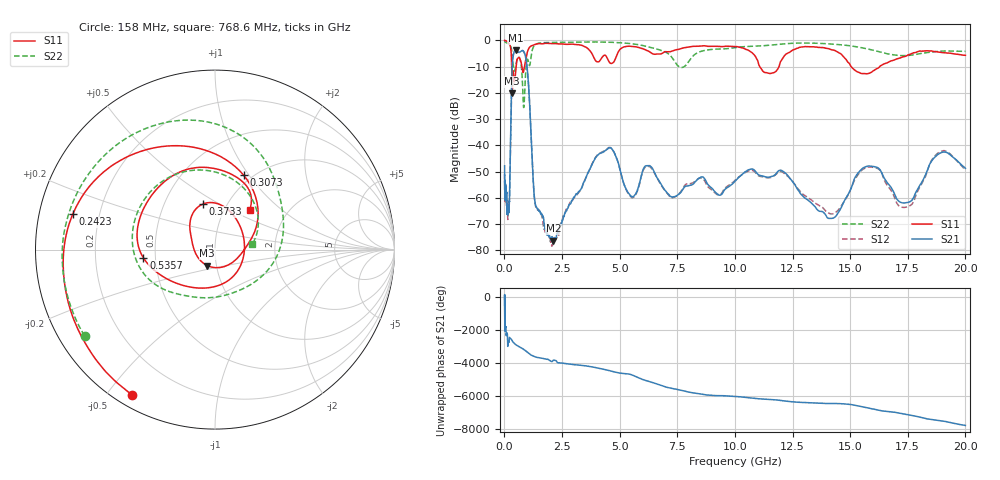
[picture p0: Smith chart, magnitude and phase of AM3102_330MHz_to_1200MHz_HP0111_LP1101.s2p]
! Date/Time: Tue, Sep 11, 2018 5:16 PM
! Network Analyzer: Agilent Technologies E8362B Rev: A.07.50.63
! Sweep from 0.010 to 20.000 GHz, 1601 Points, Sweep Type: LOG
! Power Supply: 4.949 V, 0.001 A
# Hz S DB R 50
!freq MagS11 AngS11 MagS21 AngS21 MagS12 AngS12 MagS22 AngS22
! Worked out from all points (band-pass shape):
!   1601 points, 10 MHz to 20 GHz, reference 50 ohm
!   highest |S21| = -3.69 dB at 491.8 MHz (marker M1); lowest = -76.3 dB at 2.124 GHz (marker M2)
!   |S21| within 3 dB of the highest: 368.5 MHz to 930.7 MHz (562.2 MHz wide, 86.6 % of centre)
!   lowest |S11| = -20.1 dB at 341.1 MHz (marker M3), VSWR 1.22, Z = 45.1 - j8.07 ohm
!   |S11| at or under -10 dB: 317.2 MHz to 509.5 MHz (192.2 MHz wide, 46.5 % of centre); 11.08 GHz to 11.91 GHz (831.3 MHz wide, 7.23 % of centre); 15.04 GHz to 16.28 GHz (1.234 GHz wide, 7.88 % of centre)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
!   |S22| runs from -25.6 to -0.3 dB; largest |S21 - S12| = 0.011
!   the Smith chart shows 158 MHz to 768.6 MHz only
!   S11 on the Smith chart (normalised r, x): 158 MHz: 0.05, -0.58; 242.3 MHz: 0.10, +0.12; 307.3 MHz: 0.92, +0.94; 373.3 MHz: 0.77, +0.42; 535.7 MHz: 0.43, -0.05; 768.6 MHz: 1.31, +0.64
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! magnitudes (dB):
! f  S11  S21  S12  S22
! 10 MHz  0.0  -47.8  -51.5  -0.3
! 35.55 MHz  0.0  -58.7  -59.0  -0.6
! 126.4 MHz  -0.4  -66.2  -65.6  -1.1
! 158 MHz  -0.6  -64.0  -64.8  -1.2
! 242.3 MHz  -1.8  -51.1  -51.2  -1.7
! 307.3 MHz  -7.1  -20.1  -20.1  -3.2
! 341.1 MHz  -20.1  -9.8  -9.8  -6.0
! 373.3 MHz  -11.6  -6.4  -6.4  -8.5
! 447.2 MHz  -15.1  -3.9  -3.9  -11.5
! 491.8 MHz  -11.8  -3.7  -3.8  -9.9
! 535.7 MHz  -7.9  -4.1  -4.1  -7.5
! 768.6 MHz  -10.6  -3.9  -3.9  -13.6
! 841.2 MHz  -11.5  -4.2  -4.3  -25.5
! 988.7 MHz  -4.7  -10.5  -10.6  -7.4
! 1.302 GHz  -1.6  -59.9  -60.2  -1.9
! 1.59 GHz  -1.3  -66.1  -65.7  -0.9
! 2.124 GHz  -1.2  -76.3  -76.7  -0.7
! 4.436 GHz  -6.3  -41.6  -41.4  -0.6
! 5.652 GHz  -2.4  -59.0  -59.4  -1.4
! 11.92 GHz  -10.0  -49.6  -50.0  -1.5
! 14.07 GHz  -3.1  -67.8  -65.8  -1.3
! 20 GHz  -5.7  -48.7  -49.4  -4.2
